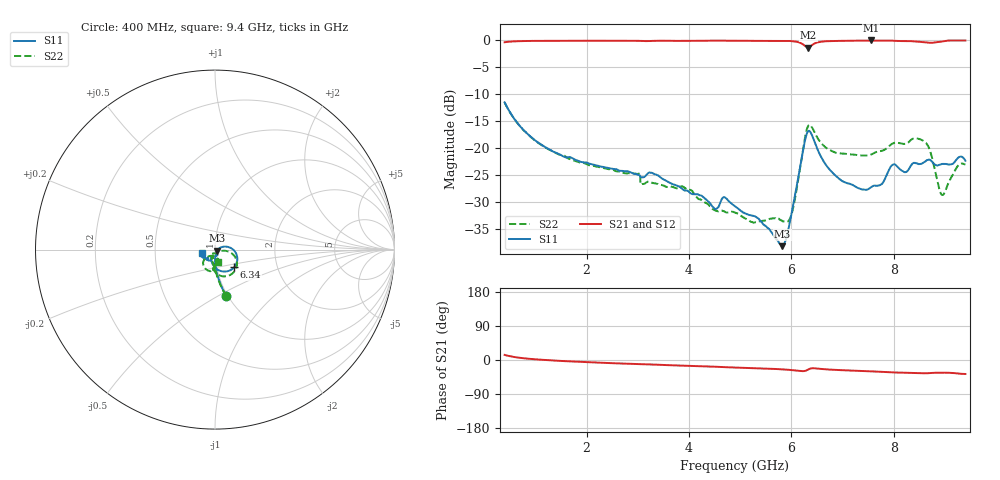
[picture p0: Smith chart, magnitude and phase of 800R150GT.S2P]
!  American Technical Ceramics  Date:  6/19/09
!  One Norden Lane
!  Huntington Station,  NY.  11746-2102
!  Tel:  (631) 622-4700  Fax:  (631) 622-4748
!  Part Number  800R150GT
!  Description: Ultra-low ESR, NPO  Mounting Orientation: Vertical
!  Application: High RF power Filters, Combiners, Matching networks,
!  Antenna, DC block, Bypass and Couplers
# GHZ S DB R 50
! Freq  |S11|  S11 Ph  |S21|  S21 Ph  |S12|  S12 Ph  |S22|  S22 Ph
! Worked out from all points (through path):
!   801 points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, 400 MHz to 9.4 GHz, reference 50 ohm
!   highest |S21| = 0.00 dB at 7.555 GHz (marker M1); lowest = -1.3 dB at 6.329 GHz (marker M2)
!   group delay of S21, straight-line fit = 12.8 ps
!   lowest |S11| = -38.1 dB at 5.823 GHz (marker M3), VSWR 1.03, Z = 51.1 - j0.559 ohm
!   |S11| at or under -10 dB: start of sweep to end of sweep
!   |S22| runs from -33.8 to -11.5 dB; largest |S21 - S12| = 0.0025
!   S11 on the Smith chart (normalised r, x): 400 MHz: 0.98, -0.55; 6.34 GHz: 1.21, -0.24; 9.4 GHz: 0.86, -0.03
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0.4  -11.48 -76.2  -0.33 13.4  -0.34 13.5  -11.49 -76.5
0.996  -18.52 -86.5  -0.08 1.9  -0.09 1.9  -18.56 -88.8
1.908  -22.54 -88.5  -0.06 -5.0  -0.06 -5.0  -22.64 -99.2
3.404  -25.05 -89.4  -0.06 -12.6  -0.06 -12.5  -26.65 -109.0
4.023  -28.25 -87.2  -0.09 -15.5  -0.09 -15.4  -27.68 -122.6
4.506  -31.22 -75.8  -0.04 -17.7  -0.04 -17.6  -31.45 -122.3
4.686  -29.06 -70.3  -0.03 -18.9  -0.04 -18.8  -31.66 -117.6
4.9  -30.74 -76.3  -0.06 -19.8  -0.06 -19.7  -31.92 -115.0
5.823  -38.13 -26.1  -0.06 -24.6  -0.06 -24.6  -33.49 -68.1
5.913  -36.29 1.8  -0.07 -25.5  -0.08 -25.4  -33.62 -52.5
6.014  -31.63 18.4  -0.13 -26.6  -0.13 -26.5  -31.91 -26.0
6.25  -19.32 -3.6  -0.89 -29.2  -0.89 -29.1  -18.89 -18.1
6.329  -16.81 -37.1  -1.31 -25.1  -1.31 -25.0  -15.84 -46.2
6.34  -16.75 -42.4  -1.28 -24.3  -1.28 -24.2  -15.71 -50.8
6.408  -17.66 -69.0  -0.83 -21.8  -0.83 -21.7  -16.17 -73.4
6.891  -25.28 -114.9  -0.09 -26.3  -0.08 -26.2  -20.86 -97.9
7.555  -27.22 -115.8  0.00 -29.9  -0.01 -29.7  -21.15 -93.0
7.904  -24.06 -111.3  -0.01 -32.3  -0.01 -32.2  -19.64 -89.9
8.613  -22.46 -137.5  -0.34 -35.0  -0.33 -34.9  -18.86 -121.6
8.95  -22.88 -145.1  -0.19 -33.5  -0.18 -33.4  -28.66 -103.8
9.254  -21.76 -147.4  -0.01 -35.7  -0.01 -35.6  -23.21 -70.8
9.4  -22.30 -165.1  -0.01 -36.9  -0.01 -36.8  -23.01 -74.6
